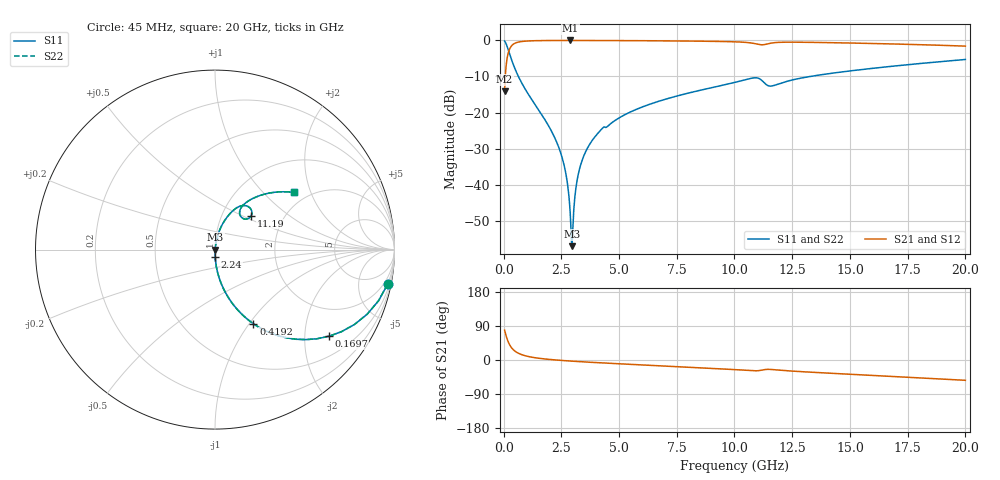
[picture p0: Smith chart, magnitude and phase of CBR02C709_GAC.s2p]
! S-parameter model data by Modelithics Inc.  support@modelithics.com 813-866-6335  Tampa FL USA
! S-Parameter data specifications:
! Substrate: 20-mil Rogers 4350B, substrate thickness, H=0.508mm, Dielectric constant, Er=3.75
! PCB Mounting Pad Footprint: Pad width, PadW=0.32mm , Pad length, PadL=0.37mm , Pad gap, PadG (edge-to-edge)=0.19mm , Reference planes=0.93mm apart
#  GHz  S  MA  R 50
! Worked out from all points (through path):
!   801 points, 45 MHz to 20 GHz, reference 50 ohm
!   highest |S21| = -0.01 dB at 2.889 GHz (marker M1); lowest = -14.1 dB at 45 MHz (marker M2)
!   group delay of S21, straight-line fit = 9.12 ps
!   lowest |S11| = -57.1 dB at 2.963 GHz (marker M3), VSWR 1.00, Z = 50.1 + j0.0225 ohm
!   |S11| at or under -10 dB: 642.6 MHz to 13.28 GHz (12.64 GHz wide, 182 % of centre)
!   |S22| runs from -57.1 to -0.2 dB; largest |S21 - S12| = 0
!   S11 on the Smith chart (normalised r, x): 45 MHz: 1, -10; 169.7 MHz: 0.99, -2.63; 419.2 MHz: 0.99, -1.05; 2.24 GHz: 1.00, -0.09; 11.19 GHz: 1.37, +0.56; 20 GHz: 1.70, +1.54
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0.045  0.9805 -11.4  0.1963 78.6  0.1963 78.6  0.9805 -11.4
0.169719  0.7971 -37.3  0.6035 52.7  0.6035 52.7  0.7971 -37.3
0.294438  0.6029 -53.2  0.7972 36.8  0.7972 36.8  0.6029 -53.2
0.419156  0.4651 -62.6  0.8845 27.3  0.8845 27.3  0.4651 -62.6
0.918031  0.2161 -78.2  0.9754 11.5  0.9754 11.5  0.2161 -78.2
2.24005  0.04298 -88.2  0.9978 0.2  0.9978 0.2  0.04298 -88.2
2.664094  0.01609 -87.1  0.9985 -1.8  0.9985 -1.8  0.01609 -87.1
2.788813  0.009116 -83.9  0.9986 -2.4  0.9986 -2.4  0.009116 -83.9
2.888587  0.003871 -72.3  0.9986 -2.8  0.9986 -2.8  0.003871 -72.3
2.963419  0.0014 9.2  0.9986 -3.1  0.9986 -3.1  0.0014 9.2
3.03825  0.004355 68.1  0.9986 -3.4  0.9986 -3.4  0.004355 68.1
3.187912  0.01163 79.1  0.9985 -3.9  0.9985 -3.9  0.01163 79.1
3.387462  0.02103 81.4  0.9983 -4.7  0.9983 -4.7  0.02103 81.4
3.736675  0.03659 81.6  0.9977 -5.9  0.9977 -5.9  0.03659 81.6
4.285437  0.06067 79.0  0.9948 -7.9  0.9948 -7.9  0.06067 79.0
6.704981  0.1428 74.1  0.9876 -15.1  0.9876 -15.1  0.1428 74.1
10.0225  0.262 62.6  0.9562 -25.5  0.9562 -25.5  0.262 62.6
11.19486  0.2769 43.1  0.8694 -26.6  0.8694 -26.6  0.2769 43.1
11.59396  0.2327 51.0  0.9176 -25.0  0.9176 -25.0  0.2327 51.0
13.36496  0.3194 56.2  0.9394 -32.4  0.9394 -32.4  0.3194 56.2
16.68248  0.4333 46.5  0.8958 -42.9  0.8958 -42.9  0.4333 46.5
20  0.5436 35.9  0.8334 -53.6  0.8334 -53.6  0.5436 35.9
